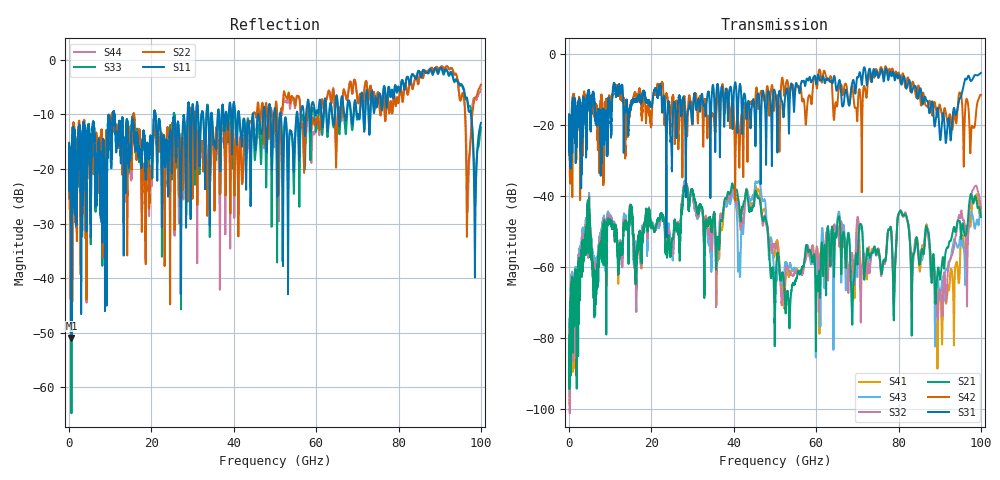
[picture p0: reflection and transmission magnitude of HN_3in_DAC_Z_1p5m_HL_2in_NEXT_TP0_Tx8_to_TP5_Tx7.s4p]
# GHz S RI R 45
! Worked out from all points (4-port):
!   4000 points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, 25 MHz to 100 GHz, reference 45 ohm
!   strongest paths, dB at 25 MHz, 25.02 GHz, 50.02 GHz, 75.03 GHz, 100 GHz:
!     S31: -17.1, -29.0, -10.7, -6.3, -5.3
!     S42: -17.1, -12.8, -11.9, -6.5, -11.5
!     S21: -89.1, -52.0, -73.4, -55.1, -45.9
!     S32: -93.6, -54.5, -54.4, -55.2, -43.6
!     S43: -91.1, -55.6, -73.7, -55.0, -43.6
!     S41: -91.9, -53.3, -55.5, -54.9, -43.4
!   lowest |S11| = -51.0 dB at 600 MHz (marker M1), VSWR 1.01, Z = 45.1 + j0.214 ohm
!   |S11| at or under -10 dB: start of sweep to 10.67 GHz; 11.03 GHz to 20.65 GHz (9.625 GHz wide, 60.8 % of centre); 20.98 GHz to 28.77 GHz (7.797 GHz wide, 31.3 % of centre)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
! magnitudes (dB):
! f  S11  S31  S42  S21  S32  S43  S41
! 25 MHz  -15.3  -17.1  -17.1  -89.1  -93.6  -91.1  -91.9
! 600 MHz  -51.0  -26.5  -24.9  -67.3  -66.9  -65.9  -66.4
! 28.3 GHz  -19.0  -31.8  -16.2  -37.6  -36.6  -36.0  -36.9
! 53.17 GHz  -42.9  -12.6  -8.4  -67.4  -60.4  -60.3  -62.0
! 80.45 GHz  -5.6  -6.9  -8.0  -44.2  -44.1  -44.1  -44.2
! 90.35 GHz  -1.5  -22.4  -16.1  -61.0  -68.3  -66.4  -71.9
! 100 GHz  -11.5  -5.3  -11.5  -45.9  -43.6  -43.6  -43.4
